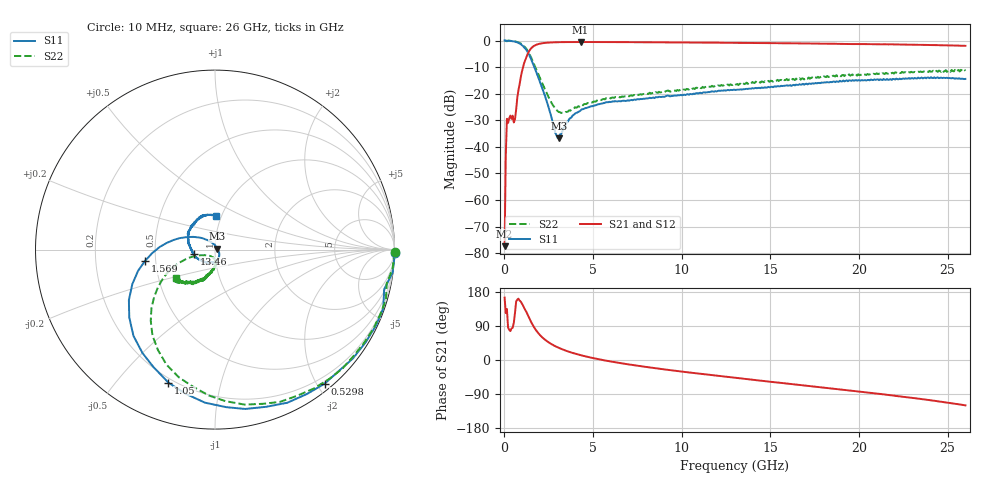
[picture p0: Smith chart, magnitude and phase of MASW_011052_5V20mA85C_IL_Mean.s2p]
! MA-COM, USA
! Part Number: MASW-011052
! Data: 29-03-2013
! Bias Condition:
!  Insertion Loss in ON stage Antenna (1) to RFin (2)
!  Forward Bias (series Diode and Shunt Diode) I = 20 mA
!  Reverse Bias Voltage V = -5V
!  Temp: 85C
!  VAR RecID: Mean
# HZ S DB R 50
! F n11x n11y n21x n21y n12x n12y n22x n22y
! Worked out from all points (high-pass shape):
!   401 points, 10 MHz to 26 GHz, reference 50 ohm
!   highest |S21| = -0.56 dB at 4.298 GHz (marker M1); lowest = -77.4 dB at 10 MHz (marker M2)
!   |S21| within 3 dB of the highest: 1.434 GHz to end of sweep
!   lowest |S11| = -36.8 dB at 3.064 GHz (marker M3), VSWR 1.03, Z = 51.3 + j0.562 ohm
!   |S11| at or under -10 dB: 1.686 GHz to end of sweep
!   |S22| runs from -27.2 to 0.0 dB; largest |S21 - S12| = 0.014
!   S11 on the Smith chart (normalised r, x): 10 MHz: -11, -92; 529.8 MHz: 0.10, -2.10; 1.05 GHz: 0.18, -0.69; 1.569 GHz: 0.44, -0.07; 13.46 GHz: 0.79, -0.04; 26 GHz: 0.94, +0.37
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1e7  0.02 -1.2  -77.36 164.6  -71.72 166.8  0.00 -0.8
2.0493e8  -0.06 -19.3  -30.98 85.8  -31.04 85.9  -0.07 -16.2
2.699e8  -0.07 -25.4  -29.27 79.6  -29.32 79.8  -0.10 -21.4
5.298e8  -0.31 -50.8  -30.84 98.5  -30.87 98.6  -0.25 -43.0
6.5975e8  -0.50 -64.7  -26.05 154.1  -26.07 154.3  -0.45 -54.5
7.897e8  -0.88 -79.2  -18.68 161.9  -18.70 162.1  -0.70 -66.8
1.0496e9  -2.10 -109.3  -10.09 143.5  -10.10 143.8  -1.79 -92.4
1.3095e9  -4.31 -141.7  -5.06 119.6  -5.06 119.8  -3.83 -119.6
1.5694e9  -8.07 -170.8  -2.54 94.6  -2.53 94.7  -7.35 -142.1
1.8293e9  -12.47 167.1  -1.51 75.6  -1.51 75.7  -11.39 -155.9
2.2192e9  -19.54 140.9  -0.94 56.2  -0.94 56.4  -17.35 -162.4
2.8689e9  -34.72 76.2  -0.66 36.5  -0.67 36.5  -25.74 -140.4
3.0638e9  -36.84 22.4  -0.63 32.1  -0.64 32.2  -26.88 -126.9
3.6486e9  -29.60 -43.2  -0.58 21.7  -0.59 21.7  -26.24 -98.6
4.2984e9  -26.32 -65.7  -0.56 12.7  -0.58 12.8  -24.44 -85.9
4.3633e9  -25.84 -65.5  -0.56 11.9  -0.58 12.0  -24.10 -88.2
8.7167e9  -21.18 -126.1  -0.68 -22.9  -0.69 -22.8  -19.29 -93.3
1.3005e10  -18.57 -162.7  -0.88 -46.9  -0.88 -46.8  -16.75 -106.9
1.346e10  -18.36 -168.1  -0.91 -49.4  -0.90 -49.1  -16.00 -106.9
1.7358e10  -16.09 162.9  -1.13 -69.5  -1.18 -69.3  -13.87 -119.7
2.1712e10  -14.65 131.1  -1.44 -92.7  -1.45 -92.3  -12.13 -131.2
2.6e10  -14.44 87.8  -1.99 -119.7  -2.05 -119.1  -11.41 -143.3
